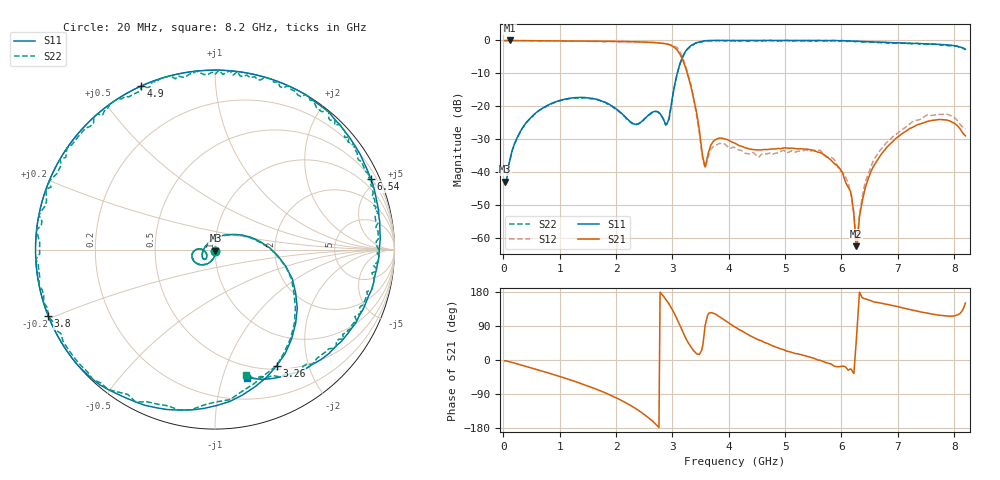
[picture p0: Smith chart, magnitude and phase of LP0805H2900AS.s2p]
!	AVX	THIN	FILM	OPERATION
!	LP0805	High	Performance	Low	Pass	Filter	P/N	LP0805H2900ASTR
!	5	February	2017
!Instrument:	"HEWLETT PACKARD,8720ES,US39172150,7.62 "
#	MHz	S	dB	R	50
!	Frq	S11(dB)	S11(deg)	S21(dB)	S21(deg)	S12(dB)	S12(deg)	S22(dB)	S22(deg)
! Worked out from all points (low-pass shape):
!   410 points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, 20 MHz to 8.2 GHz, reference 50 ohm
!   highest |S21| = -0.01 dB at 120 MHz (marker M1); lowest = -62.6 dB at 6.26 GHz (marker M2)
!   |S21| within 3 dB of the highest: start of sweep to 3.087 GHz
!   lowest |S11| = -43.0 dB at 20 MHz (marker M3), VSWR 1.01, Z = 50.2 - j0.667 ohm
!   |S11| at or under -10 dB: start of sweep to 3.085 GHz
!   |S22| runs from -43.2 to 0.0 dB; largest |S21 - S12| = 0.061
!   S11 on the Smith chart (normalised r, x): 20 MHz: 1.00, -0.01; 3.26 GHz: 0.54, -1.52; 3.8 GHz: -0.00, -0.19; 4.9 GHz: 0.00, +0.65; 6.54 GHz: 0.53, +4.57; 8.2 GHz: 0.39, -1.21
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20  -43.03 -70.1  -0.04 -2.2  -0.03 -2.1  -43.13 -70.2
120  -35.92 -81.5  -0.01 -5.2  -0.04 -5.2  -36.02 -81.5
580  -21.97 -113.5  -0.09 -24.8  -0.11 -24.8  -22.07 -113.6
1400  -17.35 -158.6  -0.19 -63.3  -0.23 -63.7  -17.55 -158.6
2180  -23.61 -178.3  -0.35 -113.6  -0.35 -113.7  -23.81 -178.3
2760  -21.99 -154.4  -0.73 -178.1  -0.74 -178.6  -22.09 -154.6
2920  -24.69 104.3  -1.18 151.9  -1.12 152.2  -24.69 104.3
3060  -11.85 10.0  -2.52 114.7  -1.98 115.3  -12.05 9.9
3260  -2.70 -62.1  -9.85 50.8  -9.26 44.0  -2.70 -62.2
3380  -1.04 -94.0  -17.96 23.9  -18.12 11.1  -1.24 -94.0
3560  -0.17 -127.3  -37.09 65.6  -37.56 57.1  -0.17 -127.3
3800  0.00 -158.2  -29.92 117.6  -31.62 113.5  0.00 -158.2
4120  0.00 170.7  -31.38 86.3  -32.83 91.6  -0.20 170.7
4900  0.00 114.2  -32.91 30.5  -33.99 43.3  0.00 114.0
5480  0.00 79.7  -33.35 6.0  -33.55 17.6  -0.10 79.7
6000  -0.05 51.4  -39.77 -16.7  -39.92 -7.0  -0.05 51.3
6160  -0.18 43.1  -45.92 -23.5  -46.21 -17.6  -0.18 43.1
6260  -0.24 38.2  -62.62 44.0  -60.21 -78.8  -0.34 38.0
6540  -0.42 24.4  -39.31 155.4  -37.71 167.9  -0.42 24.4
6840  -0.62 10.2  -31.90 146.1  -30.49 156.9  -0.82 10.0
7540  -1.05 -23.4  -24.59 123.2  -22.76 128.2  -1.05 -23.4
8200  -2.67 -75.8  -29.03 150.2  -26.99 149.1  -2.87 -75.9
